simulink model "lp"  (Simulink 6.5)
settings: Solver=ode45  StartTime=0.0  StopTime=4  RelTol=1e-3
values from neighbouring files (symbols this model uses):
  D = [J*L R*J+J*L f*R+K1*K2]    [init.m]    (also in lp4.m = @3;'))
  D1 = 0    [init.m]
  Di = [JJ*LL RR*JJ+JJ*LL K1*K2]    [init.m]
  Ds = [R*J f*R+K1*K2]    [init.m]
  Ds1 = 0    [init.m]
  I = 0    [init.m]    (also in lp4.m = @2)
  Is = 0    [init.m]
  N = Ns    (= 2)    [init.m]
  Ni = Ns    (= 2)    [init.m]
  Ns = K1    (= 2)    [init.m]
  P = 1    [init.m]
  Ps = 1    [init.m]
  Vsat = 500    [init.m]
libraries: simulink_extras x3

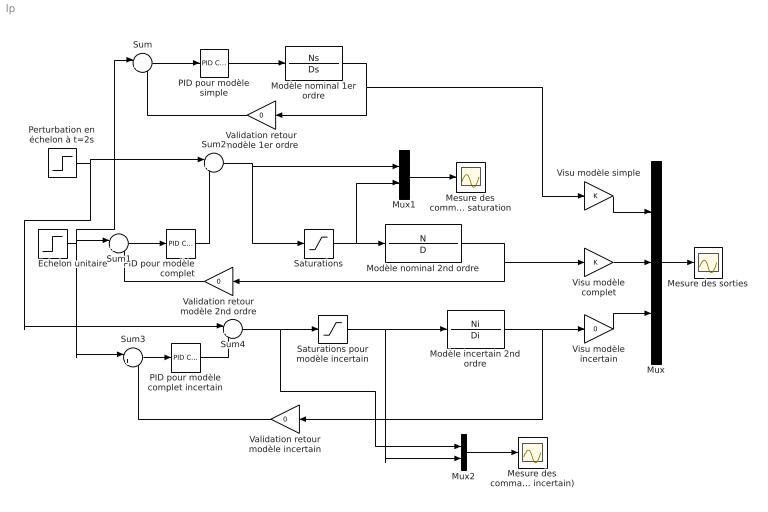
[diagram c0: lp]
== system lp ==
  Echelon unitaire : Step  Time=0  SampleTime=0
  Mesure des commandes avant et après saturation : Scope
  Mesure des commandes avant et après saturation (modèle incertain) : Scope
  Mesure des sorties : Scope
  Modèle incertain 2nd ordre : TransferFcn  Numerator=Ni  Denominator=Di
  Modèle nominal 1er ordre : TransferFcn  Numerator=Ns  Denominator=Ds
  Modèle nominal 2nd ordre : TransferFcn  Numerator=N  Denominator=D
  Mux : Mux  Inputs=3
  Mux1 : Mux  Inputs=2
  Mux2 : Mux  Inputs=2
  PID pour modèle complet : simulink_extras/Additional Linear/PID Controller  SystemSampleTime=-1  P=P  I=I  D=D1
  PID pour modèle complet incertain : simulink_extras/Additional Linear/PID Controller  SystemSampleTime=-1  P=P  I=I  D=D1
  PID pour modèle simple : simulink_extras/Additional Linear/PID Controller  SystemSampleTime=-1  P=Ps  I=Is  D=Ds1
  Perturbation en échelon à t=2s : Step  Time=2  After=0  SampleTime=0
  Saturations : Saturate  UpperLimit=Vsat  LowerLimit=-Vsat
  Saturations pour modèle incertain : Saturate  UpperLimit=Vsat  LowerLimit=-Vsat
  Sum : Sum  Inputs=|+-
  Sum1 : Sum  Inputs=|+-
  Sum2 : Sum  Inputs=|++
  Sum3 : Sum  Inputs=|+-
  Sum4 : Sum  Inputs=|++
  Validation retour modèle 1er ordre : Gain  Orientation=left  Gain=0
  Validation retour modèle 2nd ordre : Gain  Orientation=left  Gain=0
  Validation retour modèle incertain : Gain  Orientation=left  Gain=0
  Visu modèle complet : Gain
  Visu modèle incertain : Gain  Gain=0
  Visu modèle simple : Gain
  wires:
  Sum3/1 -> PID pour modèle complet incertain/1
  Validation retour modèle incertain/1 -> Sum3/2
  Mux/1 -> Mesure des sorties/1
  Sum1/1 -> PID pour modèle complet/1
  Mux1/1 -> Mesure des commandes avant et après saturation/1
  Echelon unitaire/1 -> Sum1/1, Sum3/1, Sum/1
  Validation retour modèle 2nd ordre/1 -> Sum1/2
  Sum2/1 -> Mux1/1, Saturations/1
  Perturbation en échelon à t=2s/1 -> Sum2/1, Sum4/1
  Sum/1 -> PID pour modèle simple/1
  Validation retour modèle 1er ordre/1 -> Sum/2
  Visu modèle incertain/1 -> Mux/3
  Modèle nominal 2nd ordre/1 -> Validation retour modèle 2nd ordre/1, Visu modèle complet/1
  Visu modèle complet/1 -> Mux/2
  Modèle nominal 1er ordre/1 -> Validation retour modèle 1er ordre/1, Visu modèle simple/1
  Visu modèle simple/1 -> Mux/1
  Mux2/1 -> Mesure des commandes avant et après saturation (modèle incertain)/1
  Sum4/1 -> Mux2/1, Saturations pour modèle incertain/1
  Modèle incertain 2nd ordre/1 -> Visu modèle incertain/1, Validation retour modèle incertain/1
  Saturations pour modèle incertain/1 -> Mux2/2, Modèle incertain 2nd ordre/1
  Saturations/1 -> Modèle nominal 2nd ordre/1, Mux1/2
  PID pour modèle simple/1 -> Modèle nominal 1er ordre/1
  PID pour modèle complet/1 -> Sum2/2
  PID pour modèle complet incertain/1 -> Sum4/2
